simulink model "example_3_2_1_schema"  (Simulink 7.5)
settings: Solver=ode45  StartTime=0.0  StopTime=200  FixedStep=1e-3  RelTol=1e-3
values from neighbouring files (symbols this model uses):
  A = [0 0;1 0]    [example_3_2_2_podklad.m]
  B = [7.14;0]    [example_3_2_2_podklad.m]
  C = [0 1]    [example_3_2_2_podklad.m]
  D = 0    [example_3_2_2_podklad.m]
  Kreg = lqgreg(Kalmf,K)    [example_3_2_1_podklad.m]    (also in example_3_2_2_podklad.m = lqg(sys,QXU,QWV,QXI))
  Kreg2 = lqg(sys,eye(3),QWV)    [example_3_2_1_podklad.m]
  Kreg3 = lqg(sys,0.1*eye(3),QWV,1)    [example_3_2_1_podklad.m]
  Ng = lqr_kompenzace(A,B,C,D,K)    [example_3_2_1_podklad.m]    (also in lqr_kompenzace.m = Nu + K*Nx)
undefined symbols (not defined in the file or in its folder): K, Kalmf, L
libraries: simulink x1

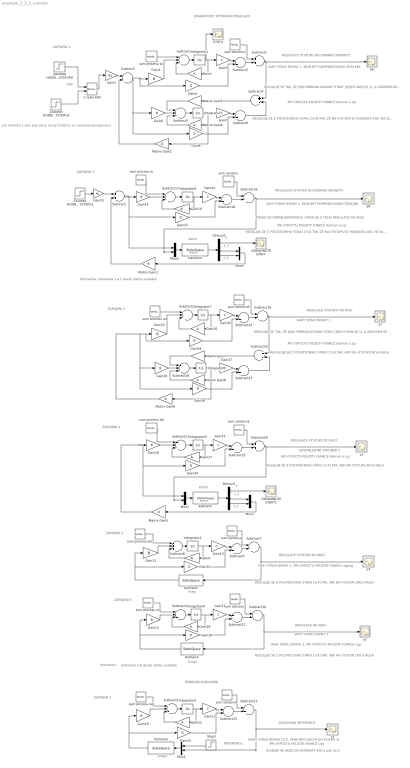
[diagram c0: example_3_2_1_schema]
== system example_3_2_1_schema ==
  note: y
  note: x_1
  note: x_2
  note: Kreg
  note: Kreg2
  note: Kreg3
  note: Kalmf
  note: REGULACE VYSTUPU DO NULY
  note: REGULACE DO NULY
  note: SLEDOVANI REFERENCE
  note: (VAHY STAVU ROVNA 1/10, VAHA REG.ODCHYLKY ROVNA 1)
  note: VAHY STAVU ROVNY 1.
  note: VAHY STAVU ROVNY 1. PRI VYPOCTU POUZITA FUNKCE Lqgreg
  note: REGULACE VYSTUPU DO ZADANE HODNOTY
  note: POKUD SE ODPOJI REFERENCE, STAVA SE Z TOHO REGULACE DO NULY
  note: REGULACE VYSTUPU DO ZADANE HODNOTY
  note: VAHY STAVU ROVNY 1. MUSI BYT KOMPENZOVANO ZESILENI.
  note: ZAPOJENI 1
  note: ZAPOJENI 2
  note: ZAPOJENI 5
  note: ZAPOJENI 6
  note: ZAPOJENI 7
  note: REFERENCE
  note: REGULUJE SE TAK, ZE JSOU MINIMALIZOVANY STAVY (JEJICH VAHA JE 1), A ZAROVEN SE VYSTUP USTALI NA ZADANE HODNOTE. TOHO JE DOCILENO SKRZ KOMPENZACI ZESILENI Ng ZAPOJENI DAVA STEJNY VYSLEDEK JAKO ZAPOJENI 2. POKUD SE ODPOJI REFERENCE, STAVA SE Z TOHO REGULACE DO NULY.
  note: KVADRATICKY OPTIMALNI REGULACE
  note: PROBLEM SLEDOVANI
  note: y
  note: x_1
  note: x_2
  note: Kalmf
  note: REGULACE VYSTUPU DO NULY
  note: EKVIVALENTNI ZAPOJENI 3
  note: REGULACE VYSTUPU DO NULY
  note: VAHY STAVU ROVNY 1.
  note: ZAPOJENI 3
  note: ZAPOJENI 4
  note: REGULUJE SE TAK, ZE JSOU MINIMALIZOVANY STAVY (JEJICH VAHA JE 1), A ZAROVEN SE VYSTUP USTALI NA NULE.
  note: PRI VYPOCTU POUZITY FUNKCE Kalman a Lqr
  note: PRI VYPOCTU POUZITY FUNKCE Kalman a Lqr
  note: PRI VYPOCTU POUZITY FUNKCE Kalman a Lqr
  note: PRI VYPOCTU POUZITY FUNKCE Kalman a Lqr
  note: VAHY STAVU ROVNY 1. PRI VYPOCTU POUZITA FUNKCE Lqg
  note: PRI VYPOCTU POUZITA FUNKCE Lqg
  note: REGULUJE SE Z POCATECNIHO STAVU [3;4] TAK, ZE NA VYSTUPU JE HODNOTA 400. VIZ BLOK ZADANA HODNOTA NA VYSTUPU
  note: REGULUJE SE Z POCATECNIHO STAVU [3;4] TAK, ABY NA VYSTUPU BYLA NULA
  note: REGULUJE SE Z POCATECNIHO STAVU [3;4] TAK, ZE NA VYSTUPU JE HODNOTA 400. VIZ BLOK ZADANA HODNOTA NA VYSTUPU
  note: REGULUJE SE Z POCATECNIHO STAVU [3;4] TAK, ABY NA VYSTUPU BYLA NULA
  note: REGULUJE SE Z POCATECNIHO STAVU [3;4] TAK, ABY NA VYSTUPU BYLA NULA
  note: REGULUJE SE Z POCATECNIHO STAVU [3;4] TAK, ABY NA VYSTUPU BYLA NULA
  note: schemata 3-6 davaji stejny vysledek
  note: Poznamka:
  note: Poznamka: schemata 1 a 2 davaji stejny vysledek
  note: VAHY STAVU ROVNY 1. MUSI BYT KOMPENZOVANO ZESILENI.
  note: SLEDUJE SE SKOK DO HODNOTY 400 a pak na 0
  note: pro hodnotu 1 jsou pak stavy rovny [0,56;0], viz odvozeni kompenzace
  note: 400
  note: Kalmf
  note: Kalmf
  0,56 0 : Scope
  1 nebo 400 : simulink/Signal Routing/Manual Switch  SystemSampleTime=-1  sw=0  action=0  varsize=off
  Demux1 : Demux  Outputs=3
  Demux2 : Demux  Outputs=3
  Gain{1,9..10,18,22,26..27} (7 alike) : Gain  Gain=A  Multiplication=Matrix(K*u)  ParameterDataType=sfix(16)  ParameterScaling=2^0  OutDataType=sfix(16)  OutScaling=2^0
  Gain{3,6,11,14..15,19,28,33,36} (9 alike) : Gain  Gain=B  Multiplication=Matrix(K*u)  ParameterDataType=sfix(16)  ParameterScaling=2^0  OutDataType=sfix(16)  OutScaling=2^0
  Gain{4,8,12,16,20,23,30,34,38} (9 alike) : Gain  Gain=D  Multiplication=Matrix(K*u)  ParameterDataType=sfix(16)  ParameterScaling=2^0  OutDataType=sfix(16)  OutScaling=2^0
  Gain{5,7,13,17,21,24,31,35,37} (9 alike) : Gain  Gain=C  Multiplication=Matrix(K*u)  ParameterDataType=sfix(16)  ParameterScaling=2^0  OutDataType=sfix(16)  OutScaling=2^0
  Gain2 : Gain  Gain=Ng  ParameterDataType=sfix(16)  ParameterScaling=2^0  OutDataType=sfix(16)  OutScaling=2^0
  Gain25 : Gain  Gain=Ng  ParameterDataType=sfix(16)  ParameterScaling=2^0  OutDataType=sfix(16)  OutScaling=2^0
  Integrator{1..2,4..7,9} (7 alike) : Integrator  InitialCondition=[3;4]
  Integrator3 : Integrator
  Integrator8 : Integrator
  Kalman1 : StateSpace  A=Kreg2.a  B=Kreg2.b  C=Kreg2.c  D=Kreg2.d
  Kalman2 : StateSpace  A=Kreg.a  B=Kreg.b  C=Kreg.c  D=Kreg.d
  Kalman3 : StateSpace  A=Kreg3.a  B=Kreg3.b  C=Kreg3.c  D=Kreg3.d
  Kalman4 : StateSpace  A=Kalmf.a  B=Kalmf.b  C=Kalmf.c  D=Kalmf.d
  Kalman5 : StateSpace  A=Kalmf.a  B=Kalmf.b  C=Kalmf.c  D=Kalmf.d
  Matrix Gain{1..2,5..6} (4 alike) : Gain  Gain=-K  Multiplication=Matrix(K*u)  ParameterDataType=sfix(16)  ParameterScaling=2^0  OutDataType=sfix(16)  OutScaling=2^0
  Matrix Gain3 : Gain  Gain=L  Multiplication=Matrix(K*u)  ParameterDataType=sfix(16)  ParameterScaling=2^0  OutDataType=sfix(16)  OutScaling=2^0
  Matrix Gain4 : Gain  Gain=A  Multiplication=Matrix(K*u)  ParameterDataType=sfix(16)  ParameterScaling=2^0  OutDataType=sfix(16)  OutScaling=2^0
  Matrix Gain7 : Gain  Gain=L  Multiplication=Matrix(K*u)  ParameterDataType=sfix(16)  ParameterScaling=2^0  OutDataType=sfix(16)  OutScaling=2^0
  Matrix Gain8 : Gain  Gain=A  Multiplication=Matrix(K*u)  ParameterDataType=sfix(16)  ParameterScaling=2^0  OutDataType=sfix(16)  OutScaling=2^0
  Mux{1..3,5..6} (5 alike) : Mux  Inputs=2
  ODHADNUTE STAVY : Scope
  ODHADNUTE STAVY1 : Scope
  Step3 : Step  Time=50  Before=400  After=0  SampleTime=0
  Subtrac2 : Sum  OutDataType=sfix(16)  OutScaling=2^-10
  Subtrac5 : Sum  OutDataType=sfix(16)  OutScaling=2^-10
  Subtract{1,3,6..7,9..10,12..13,15..16,18..20,22,24,27} (16 alike) : Sum  OutDataType=sfix(16)  OutScaling=2^-10
  Subtract{2,5,8,11,14,17,21,23,26} (9 alike) : Sum  Inputs=+++  OutDataType=sfix(16)  OutScaling=2^-10
  Subtract25 : Sum  Inputs=+-  OutDataType=sfix(16)  OutScaling=2^-10
  Subtract4 : Sum  Inputs=+-  OutDataType=sfix(16)  OutScaling=2^-10
  ZADANA HODNOTA VYSTUPU : Step  Time=0  After=400  SampleTime=0
  ZADANA HODNOTA VYSTUPU1 : Step  Time=0  After=400  SampleTime=0
  ZADANA HODNOTA VYSTUPU2 : Step  Time=0  SampleTime=0
  sum procesu w{,1..6} (7 alike) : RandomNumber  Variance=0.02  SampleTime=0
  sum senzoru{,1..6} (7 alike) : RandomNumber  Variance=0.02  SampleTime=0
  y{1..4,6..8} (7 alike) : Scope
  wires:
  sum senzoru1/1 -> Subtract1/1
  Integrator1/1 -> Gain5/1, Gain1/1, 0,56 0/1
  Subtract2/1 -> Integrator1/1
  Subtract3/1 -> Subtract1/2
  Subtract1/1 -> Subtract4/1, y6/1
  Gain5/1 -> Subtract3/1
  Gain4/1 -> Subtract3/2
  Gain1/1 -> Subtract2/3
  Gain3/1 -> Subtract2/2
  sum procesu w1/1 -> Subtract2/1
  Gain6/1 -> Subtract5/2
  Matrix Gain3/1 -> Subtract5/1
  Subtract4/1 -> Matrix Gain3/1
  Subtract5/1 -> Integrator3/1
  Gain7/1 -> Subtract6/1
  Gain8/1 -> Subtract6/2
  Subtract6/1 -> Subtract4/2
  Matrix Gain4/1 -> Subtract5/3
  Matrix Gain2/1 -> Subtrac5/2
  Integrator2/1 -> Gain9/1, Gain13/1
  Subtract8/1 -> Integrator2/1
  Subtract9/1 -> Subtract7/2
  Gain13/1 -> Subtract9/1
  Gain12/1 -> Subtract9/2
  Gain9/1 -> Subtract8/3
  Gain11/1 -> Subtract8/2
  Subtract7/1 -> Kalman2/1, y4/1
  Kalman2/1 -> Gain11/1, Gain12/1
  Integrator4/1 -> Gain17/1, Gain18/1
  Subtract11/1 -> Integrator4/1
  Subtract12/1 -> Subtract10/2
  Gain17/1 -> Subtract12/1
  Gain16/1 -> Subtract12/2
  Gain18/1 -> Subtract11/3
  Gain15/1 -> Subtract11/2
  Subtract10/1 -> Kalman1/1, y2/1
  Kalman1/1 -> Gain15/1, Gain16/1
  Integrator5/1 -> Gain21/1, Gain22/1
  Subtract14/1 -> Integrator5/1
  Subtract15/1 -> Subtract13/2
  Gain21/1 -> Subtract15/1
  Gain20/1 -> Subtract15/2
  Gain22/1 -> Subtract14/3
  Gain19/1 -> Subtract14/2
  Mux1/1 -> Kalman3/1
  Subtract13/1 -> Mux1/2, y3/1
  Subtrac5/1 -> Gain3/1, Gain4/1, Gain6/1, Gain8/1
  Integrator3/1 -> Gain7/1, Matrix Gain4/1, Matrix Gain2/1
  sum senzoru2/1 -> Subtract7/1
  sum procesu w2/1 -> Subtract8/1
  sum senzoru3/1 -> Subtract10/1
  sum procesu w3/1 -> Subtract11/1
  sum senzoru4/1 -> Subtract13/1
  sum procesu w4/1 -> Subtract14/1
  Kalman3/1 -> Gain19/1, Gain20/1
  sum senzoru/1 -> Subtract16/1
  Integrator6/1 -> Gain24/1, Gain10/1
  Subtract17/1 -> Integrator6/1
  Subtract18/1 -> Subtract16/2
  Subtract16/1 -> Mux5/2, y8/1
  Kalman4/1 -> Demux2/1
  Mux5/1 -> Kalman4/1
  Mux6/1 -> Matrix Gain1/1
  Gain24/1 -> Subtract18/1
  Gain23/1 -> Subtract18/2
  Gain10/1 -> Subtract17/3
  Gain14/1 -> Subtract17/2
  Matrix Gain1/1 -> Subtrac2/2
  Demux2/2 -> Mux6/1
  Demux2/3 -> Mux6/2
  sum procesu w/1 -> Subtract17/1
  Subtrac2/1 -> Gain14/1, Gain23/1, Mux5/1
  ZADANA HODNOTA VYSTUPU1/1 -> Gain25/1
  Step3/1 -> Mux1/1
  Gain25/1 -> Subtrac2/1
  Gain2/1 -> Subtrac5/1
  Demux2/1 -> ODHADNUTE STAVY/1
  sum senzoru6/1 -> Subtract19/1
  Integrator7/1 -> Gain35/1, Gain26/1
  Subtract23/1 -> Integrator7/1
  Subtract24/1 -> Subtract19/2
  Subtract19/1 -> y7/1, Subtract25/1
  Gain35/1 -> Subtract24/1
  Gain34/1 -> Subtract24/2
  Gain26/1 -> Subtract23/3
  Gain33/1 -> Subtract23/2
  sum procesu w6/1 -> Subtract23/1
  Gain36/1 -> Subtract26/2
  Matrix Gain7/1 -> Subtract26/1
  Subtract25/1 -> Matrix Gain7/1
  Subtract26/1 -> Integrator8/1
  Gain37/1 -> Subtract27/1
  Gain38/1 -> Subtract27/2
  Subtract27/1 -> Subtract25/2
  Matrix Gain8/1 -> Subtract26/3
  Matrix Gain6/1 -> Gain38/1, Gain36/1, Gain34/1, Gain33/1
  Integrator8/1 -> Matrix Gain6/1, Matrix Gain8/1, Gain37/1
  sum senzoru5/1 -> Subtract20/1
  Integrator9/1 -> Gain31/1, Gain27/1
  Subtract21/1 -> Integrator9/1
  Subtract22/1 -> Subtract20/2
  Subtract20/1 -> y1/1, Mux2/2
  Kalman5/1 -> Demux1/1
  Mux2/1 -> Kalman5/1
  Mux3/1 -> Matrix Gain5/1
  Gain31/1 -> Subtract22/1
  Gain30/1 -> Subtract22/2
  Gain27/1 -> Subtract21/3
  Gain28/1 -> Subtract21/2
  Matrix Gain5/1 -> Mux2/1, Gain30/1, Gain28/1
  Demux1/2 -> Mux3/1
  Demux1/3 -> Mux3/2
  sum procesu w5/1 -> Subtract21/1
  Demux1/1 -> ODHADNUTE STAVY1/1
  ZADANA HODNOTA VYSTUPU/1 -> 1 nebo 400/1
  ZADANA HODNOTA VYSTUPU2/1 -> 1 nebo 400/2
  1 nebo 400/1 -> Gain2/1
